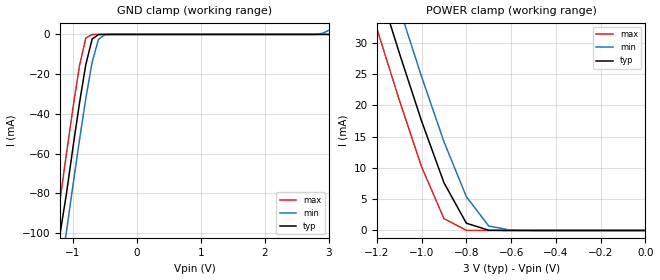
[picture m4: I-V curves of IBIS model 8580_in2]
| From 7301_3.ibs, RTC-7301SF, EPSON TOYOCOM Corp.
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|   Model 8580_in2
[Model]   8580_in2
Model_type   Input
Vinl =   0.60V
Vinh =   2.40V
C_comp   8.00pF   8.00pF   8.00pF
[Temperature Range]   25.00   85.00   -40.00
[Voltage Range]   3.00V   2.40V   3.60V
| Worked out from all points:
|   GND clamp passes 1 mA (typ) near -0.64 V on its own axis
|   POWER clamp passes 1 mA (typ) near -0.79 V on its own axis
[GND_clamp]
| voltage   I(typ)   I(min)   I(max)
-3V       -540mA     -560mA     -520mA
-1.3V     -130mA     -150mA     -110mA
-1.2V     -100mA     -120mA     -82.91mA
-1.1V     -79.74mA   -98.87mA   -59.57mA
-1V       -56.91mA   -75.91mA   -36.97mA
-900mV    -35.02mA   -53.6mA    -16.13mA
-800mV    -15.33mA   -32.47mA   -1.89mA
-700mV    -2.36mA    -13.97mA   -18.95uA
-600mV    -68.66uA   -2.44mA    -130nA
-500mV    -1.41uA    -130uA     -910pA
2.8V      2.64pA     38.98uA    2pA
3V        3.08pA     2mA        2.4pA
[POWER_clamp]
| voltage   I(typ)   I(min)   I(max)
-3V       260mA      270mA      250mA
-1.2V     39.81mA    47.03mA    32.25mA
-1.1V     28.38mA    35.6mA     20.85mA
-1V       17.46mA    24.55mA    10.16mA
-900mV    7.61mA     14.16mA    1.88mA
-800mV    1.16mA     5.39mA     27.3uA
-700mV    33.67uA    710uA      190nA
-600mV    690nA      33.17uA    1.31nA
0V        3pA        14.46pA    3.6pA
